{attribute 'TcGenerated'}
// This function has been automatically generated from the project information.
VAR_GLOBAL CONSTANT
	{attribute 'const_non_replaced'}
	{attribute 'linkalways'}
	stLibVersion_ACS_TwinCAT_Library : ST_LibVersion := (iMajor := 1, iMinor := 0, iBuild := 0, iRevision := 0, sVersion := '1.0');
END_VAR
